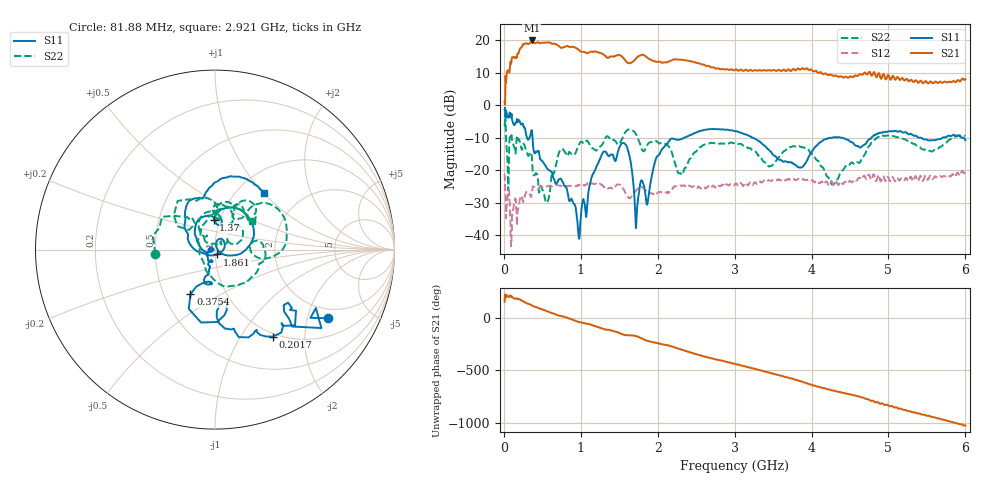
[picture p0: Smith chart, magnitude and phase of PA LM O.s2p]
!  29/10/2024  10:12:24
! Ref Plane: 0.000 mm
# MHZ S MA R  50
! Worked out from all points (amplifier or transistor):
!   1001 points, 10 MHz to 6 GHz, reference 50 ohm
!   highest |S21| = 19.9 dB at 363.4 MHz (marker M1)
!   |S21| within 3 dB of that: 202 MHz to 978.4 MHz (776.3 MHz wide, 132 % of centre)
!   unconditionally stable (mu >= 1): start of sweep to end of sweep
!   at 1.004 GHz: K = 1.34, MAG = 16.8 dB, |S12| = -24.2 dB
!   at 3.005 GHz: K = 1.93, MAG = 12.0 dB, |S12| = -24.3 dB
!   at 6 GHz: K = 1.78, MAG = 9.1 dB, |S12| = -20.5 dB
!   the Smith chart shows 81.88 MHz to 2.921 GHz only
!   S11 on the Smith chart (normalised r, x): 81.88 MHz: 1.61, -2.69; 201.7 MHz: 0.95, -1.39; 375.4 MHz: 0.68, -0.37; 1.37 GHz: 0.93, +0.32; 1.861 GHz: 1.02, -0.05; 2.921 GHz: 1.31, +1.00
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10  0.8632 4.9  1.12 154.1  0.08881 -46.1  0.4696 -81.2
81.88  0.7354 -31.4  4.195 -149.0  0.02215 -64.7  0.3335 -175.6
201.68  0.5816 -56.5  6.957 177.5  0.03205 13.7  0.2909 98.9
363.41  0.4135 -100.8  9.852 118.6  0.04426 -15.6  0.1648 20.8
375.39  0.2831 -118.9  9.431 111.6  0.05635 -25.3  0.0952 19.7
537.12  0.1201 -106.1  9.153 70.2  0.05678 -68.8  0.03474 62.1
674.89  0.06169 -111.0  8.656 31.3  0.05886 -96.8  0.1158 130.8
854.59  0.0335 -161.0  7.822 -8.2  0.05792 -130.1  0.1906 82.7
1010.33  0.02572 -150.3  6.592 -45.3  0.06055 -157.8  0.2747 73.2
1369.73  0.1657 92.4  5.459 -115.4  0.05337 135.6  0.3139 43.2
1525.47  0.2518 68.5  5.703 -153.0  0.0576 99.8  0.2839 49.6
1860.91  0.02966 -64.6  5.414 141.2  0.04699 53.3  0.2398 12.0
2010.66  0.1703 151.8  4.676 115.9  0.04606 39.5  0.2624 -16.8
2453.92  0.3593 92.3  4.619 22.9  0.05606 -34.9  0.169 105.4
2921.14  0.4163 49.3  3.486 -65.8  0.05835 -112.5  0.259 38.1
3005  0.3983 41.6  3.483 -79.2  0.06126 -124.1  0.2626 29.5
3538.11  0.1616 23.1  3.368 178.7  0.06974 139.4  0.1389 46.5
4005.33  0.1952 94.3  3.466 77.3  0.07038 49.5  0.1785 2.4
4586.36  0.2362 60.1  2.818 -27.4  0.06911 -41.2  0.131 73.9
5005.66  0.3959 64.2  2.809 -122.8  0.07378 -130.2  0.3383 51.7
5395.01  0.315 48.5  2.228 166.8  0.07195 170.8  0.2269 28.9
6000  0.2897 45.3  2.509 51.8  0.09438 61.1  0.3364 13.5
